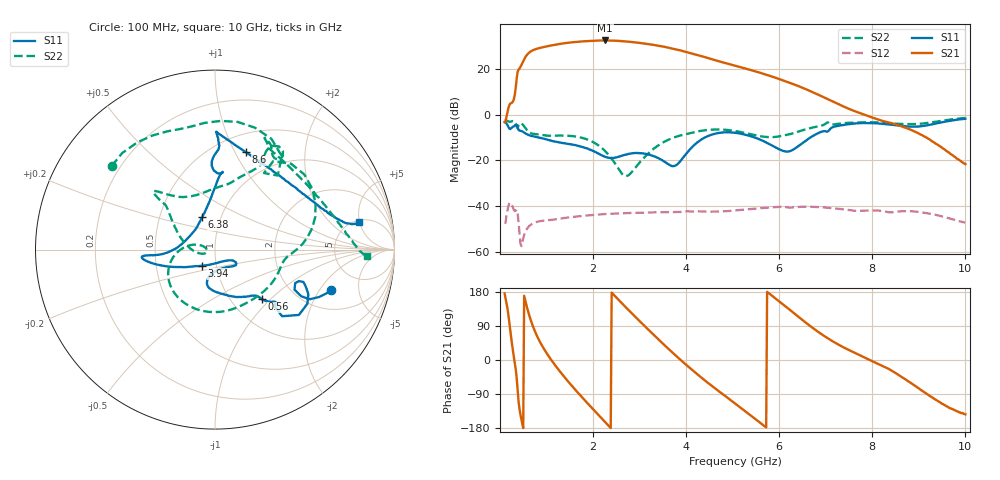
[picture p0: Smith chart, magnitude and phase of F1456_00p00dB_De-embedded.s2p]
! Integrated Device Technology
! Corporate Headquarters
! 6024 Silver Creek Valley Road
! San Jose, CA 95138  USA
! Phone:  1-408-284-8200
! Toll Free:  1-800-223-1366
! Webpage:  http://www.idt.com/
! Timing and RF Division
! 515 Groton Road, Suite 102
! Westford, MA 01886-6024
! Device:  F1456
! Description: 6-bit 0.5 dB Transmit Variable Gain Amplifier
! Frequency:  2100.0 -  2950.00 MHz
! Package:  6x6 mm Thin QFN Plastic Package: 28 pin
! State:  0
! Atten State:  0.0 dB
! Voltage:  +5.00 Volts
! Current:  213.014 mA
! Data:  The device was measured on a the F1455 evaluation board which has
!  individual transmission lines to the RF pins.  Data was collected
!  using a calibrated network analyzer.  The evaluation board was
!  de-embedded using a TRL calibration technique.
!  The reference plane is the edge of the package pin.
!  Pin  1 = CSb
!  Pin  2 = DATA
!  Pin  3 = CLK
!  Pin  4 = RSET
!  Pin  5 = GND
!  Pin  6 = RFIN  = Port 1
!  Pin  7 = GND
!  Pin  8 = NC
!  Pin  9 = NC
!  Pin 10 = NC
!  Pin 11 = NC
!  Pin 12 = NC
!  Pin 13 = NC
!  Pin 14 = /STBY
!  Pin 15 = GND
!  Pin 16 = RFOUT  = Port 2
!  Pin 17 = GND
!  Pin 18 = NC
!  Pin 19 = NC
!  Pin 20 = NC
!  Pin 21 = GND
!  Pin 22 = NC
!  Pin 23 = GND
!  Pin 24 = NC
!  Pin 25 = NC
!  Pin 26 = NC
!  Pin 27 = GND
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# GHz S dB R 50
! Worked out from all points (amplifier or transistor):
!   496 points, 100 MHz to 10 GHz, reference 50 ohm
!   highest |S21| = 32.5 dB at 2.26 GHz (marker M1)
!   |S21| within 3 dB of that: 914.2 MHz to 3.584 GHz (2.67 GHz wide, 119 % of centre)
!   unconditionally stable (mu >= 1): start of sweep to end of sweep
!   at 1.74 GHz: K = 1.98, MAG = 32.5 dB, |S12| = -44.4 dB
!   at 5.06 GHz: K = 3.85, MAG = 22.9 dB, |S12| = -41.9 dB
!   at 10 GHz: K = 136.61, MAG = -11.5 dB, |S12| = -47.3 dB
!   S11 on the Smith chart (normalised r, x): 100 MHz: 3.03, -2.56; 560 MHz: 1.38, -0.89; 3.94 GHz: 0.85, -0.16; 6.38 GHz: 0.81, +0.31; 8.6 GHz: 0.69, +1.11; 10 GHz: 5.37, +4.82
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0.1  -3.29 -19.2  -3.25 175.9  -47.17 40.6  -2.61 141.1
0.34  -4.49 -30.4  11.95 -25.0  -42.05 -140.0  -3.88 54.4
0.42  -6.99 -41.0  20.22 -129.2  -52.07 142.4  -3.89 48.4
0.56  -8.37 -46.6  25.62 148.9  -50.68 -173.3  -6.20 3.8
0.76  -9.69 -51.5  28.62 73.3  -47.19 129.4  -8.51 -19.4
0.94  -10.54 -62.6  29.59 30.4  -46.40 95.4  -9.06 -46.3
1.12  -11.52 -74.4  30.36 -2.9  -46.05 73.8  -9.24 -71.4
1.48  -12.86 -93.5  31.51 -58.9  -44.98 44.6  -9.27 -117.4
1.76  -14.12 -103.2  32.05 -98.0  -44.36 26.5  -10.13 -145.2
2.26  -18.44 -87.4  32.48 -164.0  -43.53 -1.6  -15.96 173.3
2.54  -18.43 -55.3  32.29 159.9  -43.26 -16.0  -23.51 164.5
2.86  -16.87 -37.9  31.73 119.8  -43.03 -31.6  -24.45 -160.0
3.12  -17.11 -32.6  31.09 88.3  -42.87 -43.9  -18.36 -176.9
3.4  -18.98 -32.8  30.20 55.0  -42.76 -56.7  -13.54 158.9
3.94  -18.69 -129.2  27.78 -6.3  -42.52 -79.4  -8.78 138.3
4.42  -9.82 -164.5  25.07 -55.7  -42.45 -101.4  -6.81 137.5
5.06  -7.96 -175.0  21.36 -115.4  -41.95 -125.6  -7.19 133.3
6.38  -14.23 111.8  12.76 117.3  -40.45 159.9  -7.60 72.1
6.7  -9.62 91.2  10.00 86.5  -40.34 137.8  -5.75 62.7
8.36  -4.27 82.6  -3.44 -24.0  -42.79 64.2  -3.83 62.5
8.6  -4.90 72.3  -4.91 -42.3  -42.34 58.4  -4.07 55.8
10  -1.78 10.7  -21.69 -143.4  -47.34 -17.7  -1.46 -2.5
